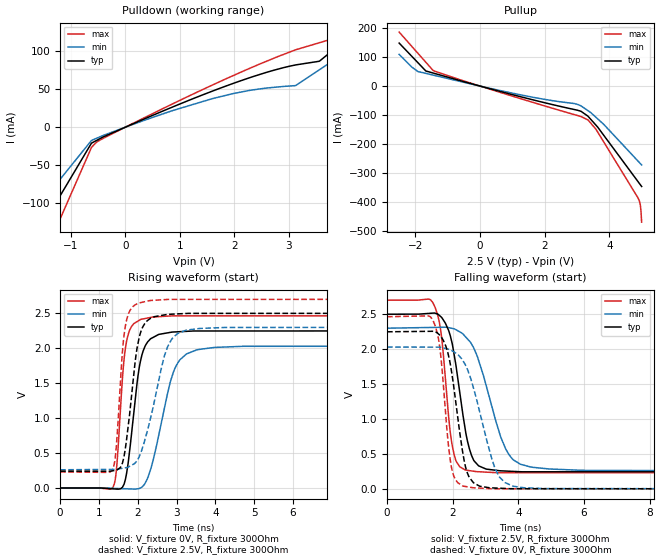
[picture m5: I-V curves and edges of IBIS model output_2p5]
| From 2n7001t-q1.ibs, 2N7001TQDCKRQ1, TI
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|   output_2p5 Model
[Model]   output_2p5
Model_type   Output
Polarity   Non-Inverting
Vmeas = 1.25
Vref = 0
Cref = 2pF
Rref = 100000
|   typ   min   max
C_comp   1.037pF   0.744pF   1.373pF
|  Where Nom  PVT is Nominal Process,   2.5V,  27C
|   Fast PVT is Strong Process,   2.7V, -40C
|   Slow PVT is Weak Process,   2.3V, 130C
[Voltage Range]   2.5   2.3   2.7
|Junction Temperature
[Temperature Range]   27   130   -40
[Pullup Reference]   2.5   2.3   2.7
[Pulldown Reference]   0   0   0
[Power Clamp Reference]   2.5   2.3   2.7
[GND Clamp Reference]   0   0   0
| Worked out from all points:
|   slope of the pulldown table from 0 to 0.375 V, typ, clamps not added: 32.1 ohm
|   slope of the pullup table from 0 to 0.375 V, typ, clamps not added: 33.6 ohm
|   falling waveform, V_fixture 2.5V, R_fixture 300Ohm: 20-80 % time 449ps typ, 778ps min, 299ps max; typ from 2.5 V to 0.241 V
|   rising waveform, V_fixture 0V, R_fixture 300Ohm: 20-80 % time 292ps typ, 501ps min, 193ps max; typ from 0 V to 2.25 V
|   rising waveform, V_fixture 2.5V, R_fixture 300Ohm: 20-80 % time 288ps typ, 516ps min, 188ps max; typ from 0.241 V to 2.5 V
|   falling waveform, V_fixture 0V, R_fixture 300Ohm: 20-80 % time 412ps typ, 694ps min, 284ps max; typ from 2.25 V to 0 V
[Pulldown]
|   Voltage   I(typ)   I(min)   I(max)
-2.5V     -310.2mA   -241.2mA   -1.829A
-2.182V   -256.4mA   -198.2mA   -305.8mA
-1.308V   -108.3mA   -79.74mA   -138.3mA
-1.273V   -102.5mA   -75.06mA   -132.7mA
-624.9mV  -21.09mA   -17.53mA   -26.75mA
-441.5mV  -14.09mA   -11.9mA    -15.94mA
1.584V    47.06mA    37.25mA    55mA
3.125V    81.92mA    54.7mA     101.8mA
3.561V    86.76mA    75.5mA     111.1mA
4.18V     122.6mA    105mA      148.1mA
4.279V    134.6mA    109.7mA    159.9mA
5V        221.6mA    192.7mA    245.6mA
[Pullup]
|   Voltage   I(typ)   I(min)   I(max)
-2.5V     147.7mA    109.1mA    185.5mA
-1.92V    80.36mA    49.93mA    112.7mA
-1.675V   51.79mA    43.52mA    81.83mA
-1.444V   44.57mA    37.51mA    52.91mA
1.241V    -36.28mA   -29.9mA    -42.78mA
2.915V    -80.66mA   -60.13mA   -98.1mA
3.345V    -104.3mA   -85.06mA   -116.7mA
3.59V     -134.8mA   -107.7mA   -149mA
4.883V    -327.7mA   -257.4mA   -383.6mA
4.96V     -339.3mA   -266.5mA   -409mA
4.982V    -342.5mA   -269.1mA   -431.8mA
5V        -345.3mA   -271.3mA   -468mA
[Ramp]
R_load = 300
|   typ   min   max
dV/dt_r   1.34921/2.90831e-10   1.21841/4.97647e-10   1.47857/1.91779e-10
dV/dt_f   1.35567/4.48672e-10   1.22424/7.71701e-10   1.48241/2.98374e-10
[Falling Waveform]
V_fixture = 2.5V
V_fixture_min = 2.3V
V_fixture_max = 2.7V
R_fixture = 300Ohm
C_fixture = 0F
|   Time   V(typ)   V(min)   V(max)
0s        2.5V       2.3V       2.7V
1.386ns   2.515V     2.311V     2.672V
1.631ns   2.468V     2.313V     2.282V
1.777ns   2.372V     2.314V     1.581V
2.093ns   1.786V     2.28V      414.2mV
2.413ns   768.4mV    2.165V     271.5mV
2.72ns    368.7mV    1.931V     250.7mV
3.705ns   256.9mV    500.2mV    235.4mV
4.936ns   248.2mV    288.5mV    235.3mV
40ns      240.6mV    259.6mV    229.3mV
[Rising Waveform]
V_fixture = 0V
V_fixture_min = 0V
V_fixture_max = 0V
R_fixture = 300Ohm
C_fixture = 0F
|   Time   V(typ)   V(min)   V(max)
0s        -59.5nV    164nV      -4.666nV
1.36ns    -12.26mV   -5.241mV   7.769mV
1.46ns    -15.92mV   -7.177mV   313.4mV
1.607ns   10.6mV     -10.03mV   1.577V
1.778ns   472mV      -13.34mV   2.235V
2.067ns   1.803V     -872uV     2.406V
2.394ns   2.151V     390.3mV    2.444V
3.001ns   2.231V     1.757V     2.46V
3.978ns   2.244V     2.009V     2.46V
40ns      2.249V     2.031V     2.464V
[Rising Waveform]
V_fixture = 2.5V
V_fixture_min = 2.3V
V_fixture_max = 2.7V
R_fixture = 300Ohm
C_fixture = 0F
|   Time   V(typ)   V(min)   V(max)
0s        240.6mV    259.6mV    229.3mV
1.348ns   244.7mV    265.6mV    257.9mV
1.442ns   253.9mV    266mV      554.7mV
1.573ns   311.1mV    278.2mV    1.686V
1.765ns   933.2mV    302.1mV    2.495V
2.041ns   2.159V     450.9mV    2.645V
2.319ns   2.42V      973.7mV    2.679V
2.862ns   2.484V     2.114V     2.695V
3.611ns   2.495V     2.28V      2.695V
40ns      2.5V       2.3V       2.7V
[Falling Waveform]
|Gnd
V_fixture = 0V
V_fixture_min = 0V
V_fixture_max = 0V
R_fixture = 300Ohm
C_fixture = 0F
|   Time   V(typ)   V(min)   V(max)
0s        2.249V     2.031V     2.464V
1.321ns   2.256V     2.029V     2.463V
1.568ns   2.218V     2.029V     2.147V
1.717ns   2.123V     2.016V     1.482V
1.986ns   1.614V     1.976V     259.3mV
2.35ns    405.3mV    1.805V     40.78mV
2.622ns   97.74mV    1.463V     20.4mV
3.293ns   16.46mV    290.8mV    6.053mV
4.155ns   6.687mV    20.86mV    6.027mV
40ns      6.237nV    195.7nV    37.17nV
